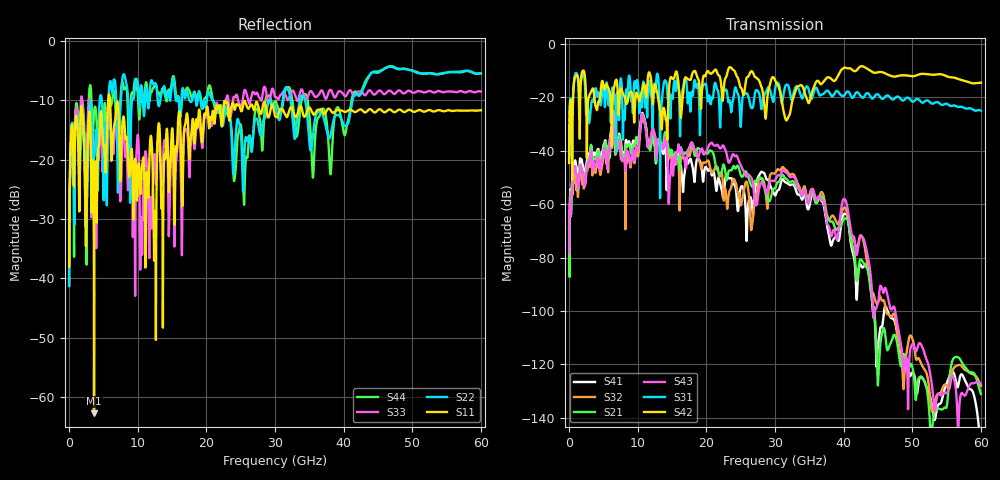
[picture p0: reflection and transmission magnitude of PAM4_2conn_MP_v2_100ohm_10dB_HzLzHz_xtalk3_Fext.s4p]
! Info: Touchstone file created by Circ.  Input file=FAB50GbE_2conn_Midplane_Examax_Topo2_v2_100ohm_10dB_HzLzHz.circ
# Hz S RI R 50
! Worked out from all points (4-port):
!   6000 points, 10 MHz to 60 GHz, reference 50 ohm
!   strongest paths, dB at 10 MHz, 15.01 GHz, 30.01 GHz, 45.01 GHz, 60 GHz:
!     S42: -44.6, -12.9, -13.6, -10.6, -14.5
!     S31: -43.6, -19.8, -17.2, -18.9, -25.0
!     S43: -78.4, -42.8, -51.2, -96.8, -127.4
!     S21: -64.7, -41.9, -54.1, -127.6, -131.1
!     S32: -69.2, -43.2, -48.5, -97.0, -128.1
!     S41: -68.5, -40.6, -56.7, -113.0, -153.8
!   lowest |S11| = -62.7 dB at 3.64 GHz (marker M1), VSWR 1.00, Z = 49.9 - j0.0433 ohm
!   |S11| at or under -10 dB: start of sweep to 5.706 GHz; 5.955 GHz to end of sweep
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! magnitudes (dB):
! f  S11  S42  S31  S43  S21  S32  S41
! 10 MHz  -38.0  -44.6  -43.6  -78.4  -64.7  -69.2  -68.5
! 3.64 GHz  -62.7  -18.9  -21.0  -44.9  -42.9  -47.0  -41.2
! 10.78 GHz  -19.8  -15.8  -14.4  -27.4  -26.7  -28.1  -26.4
! 26.62 GHz  -10.7  -10.2  -24.0  -50.4  -53.3  -68.6  -59.5
! 31.21 GHz  -11.7  -24.7  -19.4  -47.3  -49.2  -46.2  -50.8
! 41.93 GHz  -11.9  -9.8  -18.1  -78.9  -88.6  -76.9  -95.3
! 60 GHz  -11.7  -14.5  -25.0  -127.4  -131.1  -128.1  -153.8
